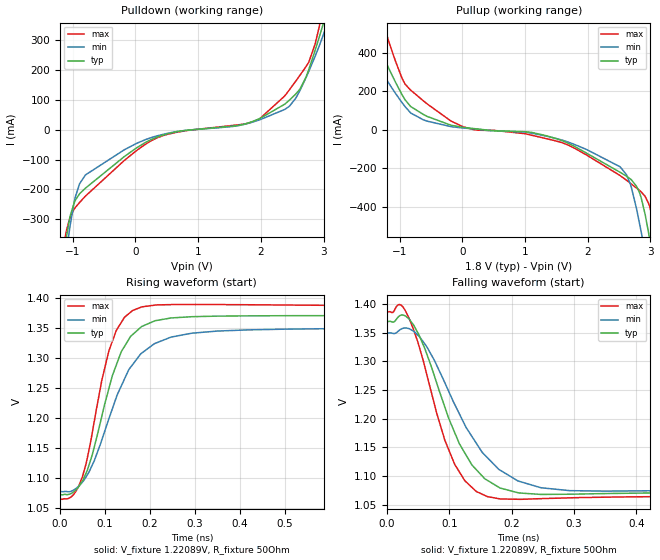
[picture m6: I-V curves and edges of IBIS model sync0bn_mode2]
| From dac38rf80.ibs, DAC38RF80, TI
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|   sync0bn_mode2 Model
[Model]   sync0bn_mode2
Model_type   Output
Polarity   Non-Inverting
Vmeas = 1.22089
Vref = 1.22089
Cref = 2pF
Rref = 200
|   typ   min   max
|   (nom PVT)   (fast PVT)   (slow PVT)
C_comp   6.095e-13   6.095e-13   6.288e-13
| Where nom  PVT is Nominal Process, 1.8V, 27C
|   Fast PVT is Strong Process,  1.89V, -40C
|   Slow PVT is Weak Process,   1.71V, 105C
[Voltage Range]   1.8   1.71   1.89
|Junction Temperature
[Temperature Range]   27   105   -40
[Pullup Reference]   1.8   1.71   1.89
[Pulldown Reference]   0   0   0
[Power Clamp Reference]   1.8   1.71   1.89
[GND Clamp Reference]   0   0   0
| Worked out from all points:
|   slope of the pulldown table from 0 to 0.27 V, typ, clamps not added: 8.35 ohm
|   slope of the pullup table from 0 to 0.27 V, typ, clamps not added: 27.1 ohm
|   falling waveform, V_fixture 1.22089V, R_fixture 50Ohm: 20-80 % time 64.8ps typ, 82.5ps min, 52.7ps max; typ from 1.37 V to 1.07 V
|   rising waveform, V_fixture 1.22089V, R_fixture 50Ohm: 20-80 % time 67.3ps typ, 90.2ps min, 54.1ps max; typ from 1.07 V to 1.37 V
[Pulldown]
|   Voltage   I(typ)   I(min)   I(max)
-1.8V     -1.67A     -1.574A    -1.834A
-1.094V   -352.6mA   -401.7mA   -333.3mA
-975.6mV  -245.1mA   -242.6mA   -266.1mA
-796.2mV  -196.1mA   -151.7mA   -222.7mA
18.18mV   -60.96mA   -46mA      -70.01mA
1.863V    27.24mA    25.3mA     25.95mA
2.381V    85.82mA    68.15mA    113.5mA
2.623V    136mA      131.2mA    182.6mA
2.762V    200.9mA    195.2mA    226.1mA
2.928V    308.8mA    279.7mA    343mA
3.084V    417.9mA    369.4mA    512.5mA
3.6V      893.4mA    1.265A     1.198A
[Pullup]
|   Voltage   I(typ)   I(min)   I(max)
-1.8V     838mA      987.9mA    1.234A
-1.6V     623.6mA    536.8mA    970.8mA
-1.306V   411.1mA    311mA      596.1mA
-815.4mV  118.7mA    85.32mA    203.1mA
6.84mV    12.6mA     8.943mA    16.65mA
1.114V    -14.44mA   -18.18mA   -29.16mA
1.976V    -120.4mA   -101.8mA   -130mA
2.617V    -240.6mA   -232.7mA   -261.4mA
2.851V    -351mA     -527.2mA   -321.5mA
2.97V     -533.5mA   -723mA     -381.7mA
3.118V    -813.8mA   -968.4mA   -610.5mA
3.6V      -1.728A    -1.772A    -1.696A
[Ramp]
R_load = 50
|   typ   min   max
dV/dt_r   0.0830373/1.59286e-10  0.0836466/1.70781e-10   0.404627/1.40143e-10
dV/dt_f   0.178314/6.47857e-11   0.163295/8.24947e-11   0.192861/5.27497e-11
[Falling Waveform]
V_fixture = 1.22089V
V_fixture_min = 1.21341V
V_fixture_max = 1.22551V
R_fixture = 50Ohm
|   Time   V(typ)   V(min)   V(max)
0s        1.369V     1.349V     1.386V
22.12ps   1.38V      1.356V     1.398V
42.68ps   1.363V     1.353V     1.355V
92.87ps   1.22V      1.263V     1.162V
108.6ps   1.176V     1.225V     1.12V
136.1ps   1.12V      1.169V     1.081V
161.3ps   1.093V     1.132V     1.064V
209.8ps   1.071V     1.092V     1.06V
293.2ps   1.068V     1.075V     1.062V
1.197ns   1.072V     1.077V     1.065V
[Rising Waveform]
V_fixture = 1.22089V
V_fixture_min = 1.21341V
V_fixture_max = 1.22551V
R_fixture = 50Ohm
|   Time   V(typ)   V(min)   V(max)
0s        1.072V     1.077V     1.065V
29.83ps   1.077V     1.08V      1.072V
49.49ps   1.095V     1.093V     1.102V
92.87ps   1.203V     1.164V     1.263V
124.9ps   1.288V     1.234V     1.346V
156.8ps   1.336V     1.285V     1.376V
181.8ps   1.353V     1.308V     1.385V
246.9ps   1.367V     1.335V     1.389V
349.8ps   1.37V      1.345V     1.389V
1.605ns   1.37V      1.35V      1.386V
